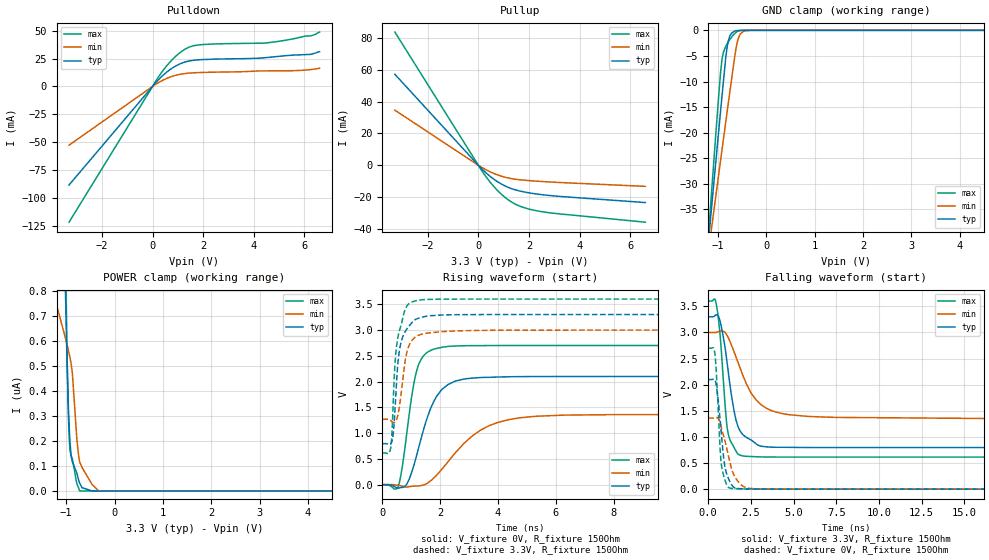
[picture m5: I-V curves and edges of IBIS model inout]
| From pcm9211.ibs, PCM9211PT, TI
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|   inout Model
[Model]   inout
Model_type   I/O
Polarity   Non-Inverting
Enable   Active-Low
Vinl = 0.8
Vinh = 2.0
Vmeas = 1.65
Vref = 0
Cref = 20pF
Rref = 200
|   typ   min   max
|   (nom PVT)   (fast PVT)   (slow PVT)
C_comp   7.115e-13   6.715e-13   7.422e-13
| Where nom  PVT is Nominal Process, 3.3V, 27C
|   Fast PVT is Strong Process,  3.6V, -40C
|   Slow PVT is Weak Process,   3V, 150C
[Voltage Range]   3.3   3   3.6
|Junction Temperature
[Temperature Range]   27   150   -40
[Pullup Reference]   3.3   3   3.6
[Pulldown Reference]   0   0   0
[Power Clamp Reference]   3.3   3   3.6
[GND Clamp Reference]   0   0   0
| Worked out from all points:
|   slope of the pulldown table from 0 to 0.495 V, typ, clamps not added: 42.4 ohm
|   slope of the pullup table from 0 to 0.495 V, typ, clamps not added: 67.6 ohm
|   GND clamp passes 1 mA (typ) near -0.75 V on its own axis
|   falling waveform, V_fixture 3.3V, R_fixture 150Ohm: 20-80 % time 710ps typ, 1.6ns min, 417ps max; typ from 3.3 V to 0.796 V
|   rising waveform, V_fixture 0V, R_fixture 150Ohm: 20-80 % time 728ps typ, 1.49ns min, 426ps max; typ from 0 V to 2.1 V
|   rising waveform, V_fixture 3.3V, R_fixture 150Ohm: 20-80 % time 245ps typ, 276ps min, 251ps max; typ from 0.795 V to 3.3 V
|   falling waveform, V_fixture 0V, R_fixture 150Ohm: 20-80 % time 391ps typ, 670ps min, 258ps max; typ from 2.1 V to 0 V
[Pulldown]
|   Voltage   I(typ)   I(min)   I(max)
-3.3V     -88.47mA   -52.71mA   -121.9mA
186mV     4.927mA    2.834mA    6.943mA
660mV     14.64mA    8.153mA    21.22mA
1.121V    20.67mA    11.06mA    30.98mA
1.441V    22.89mA    11.97mA    35.29mA
1.767V    23.82mA    12.41mA    37.14mA
2.514V    24.57mA    12.87mA    38.22mA
4.429V    25.79mA    13.98mA    38.92mA
5.28V     27.68mA    14.1mA     41.59mA
6.053V    28.64mA    14.74mA    45.32mA
6.244V    28.83mA    15.14mA    45.39mA
6.6V      31.32mA    16.33mA    48.83mA
[GND Clamp]
|   Voltage   I(typ)   I(min)   I(max)
-3.3V     -257mA     -194.6mA   -316.3mA
-1.314V   -53.34mA   -51.75mA   -55.59mA
-1.064V   -27.92mA   -33.95mA   -23.08mA
-945.6mV  -15.94mA   -25.54mA   -8.43mA
-907.5mV  -12.16mA   -22.86mA   -5.316mA
-834.9mV  -5.192mA   -17.77mA   -3.092mA
-785.4mV  -2.121mA   -14.33mA   -2.282mA
-661.2mV  -199.5uA   -5.828mA   -714.1uA
-597mV    -46.7uA    -2.27mA    -235.2uA
-540mV    -10.84uA   -770.9uA   -53.07uA
-330mV    -21.41nA   -4.003uA   -23.33nA
6.6V      0A         0A         0A
[Pullup]
|   Voltage   I(typ)   I(min)   I(max)
-3.3V     57.13mA    34.62mA    83.66mA
141.6mV   -2.35mA    -1.382mA   -3.551mA
423mV     -6.396mA   -3.75mA    -9.72mA
660mV     -9.272mA   -5.412mA   -14.19mA
1.099V    -13.31mA   -7.678mA   -20.72mA
1.301V    -14.62mA   -8.364mA   -22.96mA
1.647V    -16.19mA   -9.095mA   -25.71mA
2.436V    -18.3mA    -10.09mA   -28.93mA
6.6V      -23.39mA   -13.21mA   -35.71mA
[POWER Clamp]
|   Voltage   I(typ)   I(min)   I(max)
-3.3V     4.368uA    2.569uA    6.447uA
-1.668V   1.943uA    1.092uA    3.039uA
-1.19V    1.318uA    736.5nA    2.096uA
-1.044V   1.037uA    630.5nA    1.49uA
-1.007V   724.4nA    602.6nA    871.9nA
-957mV    346.6nA    563.2nA    317.5nA
-927.3mV  213.4nA    537.4nA    175.9nA
-873mV    116.2nA    471.2nA    128.8nA
-780mV    71.27nA    208nA      28.45nA
-723mV    31.61nA    117nA      0A
-330mV    0A         0A         0A
6.6V      0A         0A         0A
[Ramp]
R_load = 150
|   typ   min   max
dV/dt_r   1.25932/7.27751e-10   0.816956/1.48416e-09   1.61949/4.25408e-10
dV/dt_f   1.50218/7.08752e-10   1.03591/1.6044e-09   1.79161/4.16509e-10
[Falling Waveform]
V_fixture = 3.3V
V_fixture_min = 3V
V_fixture_max = 3.6V
R_fixture = 150Ohm
|   Time   V(typ)   V(min)   V(max)
0s        3.3V       3V         3.6V
399.7ps   3.323V     2.999V     3.632V
681ps     3.231V     3.026V     3.007V
1.005ns   2.67V      2.995V     1.546V
1.128ns   2.367V     2.93V      1.139V
1.505ns   1.517V     2.639V     807.3mV
1.868ns   1.114V     2.32V      651.2mV
2.82ns    864.7mV    1.704V     620.5mV
4.701ns   800.9mV    1.427V     614.3mV
25ns      796.4mV    1.273V     614mV
[Rising Waveform]
V_fixture = 0V
V_fixture_min = 0V
V_fixture_max = 0V
R_fixture = 150Ohm
|   Time   V(typ)   V(min)   V(max)
0s        770.4pV    12.07nV    637.6pV
532.3ps   -67.5mV    -12.33mV   -54.29mV
862.1ps   28.46mV    -44.51mV   1.073V
1.079ns   355.5mV    -29.23mV   1.929V
1.267ns   743.1mV    -22.71mV   2.348V
1.637ns   1.433V     60.93mV    2.595V
2.053ns   1.843V     295.3mV    2.664V
3.398ns   2.078V     1.059V     2.698V
5.265ns   2.097V     1.325V     2.699V
25ns      2.099V     1.362V     2.699V
[Rising Waveform]
V_fixture = 3.3V
V_fixture_min = 3V
V_fixture_max = 3.6V
R_fixture = 150Ohm
|   Time   V(typ)   V(min)   V(max)
0s        794.9mV    1.267V     613.3mV
299.7ps   799mV      1.24V      754.2mV
336.5ps   856.4mV    1.223V     1.047V
380.7ps   1.013V     1.208V     1.677V
434.1ps   1.431V     1.212V     2.325V
557.1ps   2.46V      1.409V     2.912V
657.6ps   2.786V     1.801V     3.116V
830.3ps   3.006V     2.528V     3.448V
1.203ns   3.219V     2.884V     3.574V
25ns      3.3V       3V         3.6V
[Falling Waveform]
V_fixture = 0V
V_fixture_min = 0V
V_fixture_max = 0V
R_fixture = 150Ohm
|   Time   V(typ)   V(min)   V(max)
0s        2.099V     1.362V     2.699V
387.1ps   2.098V     1.364V     2.601V
478.6ps   1.975V     1.37V      2.222V
742.3ps   1.169V     1.213V     555.4mV
992.8ps   401.9mV    910.1mV    162.9mV
1.24ns    164.2mV    559.1mV    24.68mV
1.505ns   35.61mV    274.9mV    11.8mV
1.857ns   9.547mV    105.4mV    5.972mV
2.772ns   2.849mV    6.472mV    382.8uV
25ns      3.725uV    2.081uV    1.292uV
